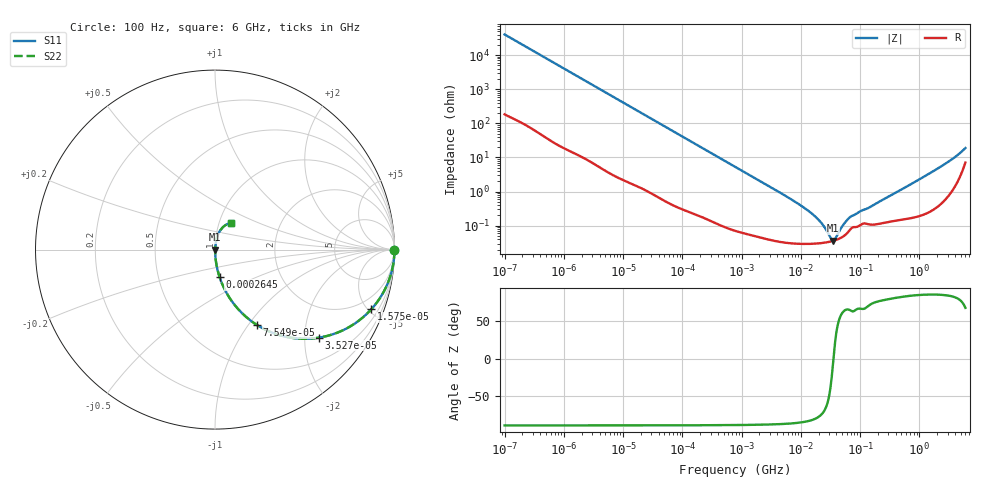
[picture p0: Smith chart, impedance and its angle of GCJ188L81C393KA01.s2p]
!Murata Part Number: GCJ188L81C393KA01
!These Parameters are Measured in Series Mode Connection
!Data Generated on Mar 13, 2026
!  o--ll--o
!Port1  Port2
!  o------o
!Operation Temp=25[degC], DC Bias Voltage=0[V]
!Freq. Start=100[Hz] Stop=6[GHz] 401[Steps]
# Hz S RI R 50
!Freq.(Hz) S11(Real) S11(Imag) S21(Real) S21(Imag) S12(Real) S12(Imag) S22(Real) S22(Imag)
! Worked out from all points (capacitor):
!   401 points, 100 Hz to 6 GHz, reference 50 ohm
!   read as one part in series: C = 39.3 nF near 109 Hz
!   lowest |Z| = 36.1 mohm at 34.83 MHz (marker M1)
!   series resonance near 35.59 MHz, so ESL is about 510 pH
!   S11 on the Smith chart (normalised r, x): 100 Hz: open; 15.75 kHz: 1.03, -5.21; 35.27 kHz: 1.02, -2.34; 75.5 kHz: 1.01, -1.09; 264.5 kHz: 1.00, -0.31; 6 GHz: 1.14, +0.35
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100  1 -0.00247  1.74e-05 0.00247  1.74e-05 0.00247  1 -0.00247
2008  0.9973 -0.0491  0.00267 0.0491  0.00267 0.0491  0.9973 -0.0491
6151  0.9772 -0.1467  0.0228 0.1467  0.0228 0.1467  0.9772 -0.1467
15752  0.8703 -0.3331  0.1297 0.3331  0.1297 0.3331  0.8703 -0.3331
35265  0.5767 -0.4909  0.4233 0.4909  0.4233 0.4909  0.5767 -0.4909
40335  0.5109 -0.4967  0.4891 0.4967  0.4891 0.4967  0.5109 -0.4967
75495  0.232 -0.4187  0.768 0.4187  0.768 0.4187  0.232 -0.4187
129199  0.095 -0.2893  0.905 0.2893  0.905 0.2893  0.095 -0.2893
264476  0.0255 -0.1529  0.9745 0.1529  0.9745 0.1529  0.0255 -0.1529
774597  0.0036 -0.0537  0.9964 0.0537  0.9964 0.0537  0.0036 -0.0537
6353432  0.000349 -0.00644  0.9997 0.00644  0.9997 0.00644  0.000349 -0.00644
1.555665e7  0.000299 -0.0022  0.9997 0.0022  0.9997 0.0022  0.000299 -0.0022
2.225763e7  0.00031 -0.00116  0.9997 0.00116  0.9997 0.00116  0.00031 -0.00116
3.184506e7  0.000343 -0.000265  0.9997 0.000265  0.9997 0.000265  0.000343 -0.000265
3.482834e7  0.000357 -5.09e-05  0.9996 5.09e-05  0.9996 5.09e-05  0.000357 -5.09e-05
3.80911e7  0.000374 0.000163  0.9996 -0.000163  0.9996 -0.000163  0.000374 0.000163
5.211241e7  0.000485 0.000941  0.9995 -0.000941  0.9995 -0.000941  0.000485 0.000941
6.817316e7  0.000772 0.00162  0.9992 -0.00162  0.9992 -0.00162  0.000772 0.00162
3.124326e8  0.00135 0.00722  0.9986 -0.00722  0.9986 -0.00722  0.00135 0.00722
2.142435e9  0.00627 0.0492  0.9937 -0.0492  0.9937 -0.0492  0.00627 0.0492
4.193612e9  0.027 0.1034  0.973 -0.1034  0.973 -0.1034  0.027 0.1034
6e9  0.0906 0.1489  0.9094 -0.1489  0.9094 -0.1489  0.0906 0.1489
